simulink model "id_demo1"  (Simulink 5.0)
settings: Solver=ode45  SolverMode=SingleTasking  StartTime=0.0  StopTime=10  RelTol=1e-3  AbsTol=1e-3
libraries: simulink x1

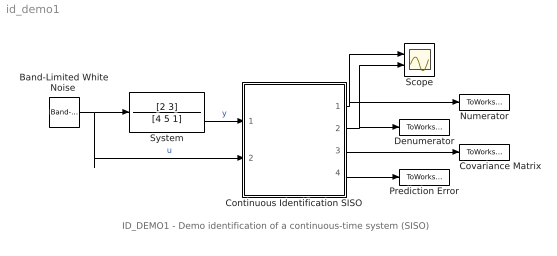
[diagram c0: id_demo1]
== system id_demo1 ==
  note: ID_DEMO1 - Demo identification of a continuous-time system (SISO)
  "Band-Limited White Noise " : simulink/Sources/Band-Limited White Noise  Cov=[0.1]  Ts=0.1  seed=[23341]
  Continuous Identification SISO : Subsystem  mask(Continuous Identification){par1=[1,2], tc=[0.5], par2=[0.985,0.01], poc=[0 0 0 0], kov=[10e6], ts=[1]}
      mask prompts: par1 "Degrees of numerator and denominator -  [dn, dd]:"; tc "Time constant of the filter - [Tc]:"; par2 "Exponential forgetting and Bittanti's correction - [L, d]:"; poc "Initial parameter estimates - [theta(1) ... theta(n)]:"; kov "Covariance matrix (see help, standard - [10e6]):"; ts "Sampling time - [ts]:"
      mask help: Continuous identification Authors: Lubos Cirka and Miroslav Fikar 1998 - 2006
      mask init:
      | % State-space realisation of continuous-time MIMO filters
      | %
      | % Input:
      | %    y1(t), ..., yn(t), u1(t), ..., um(t)
      | % Output:
      | %    y(t), y'(t), y''(t) ..., u(t), u'(t), ...
      | 
      | % Calculation of the denominator with multiple time constant tc
      | 
      | cit=par1(1);men=par1(2);L=par2(1);d=par2(2); n=cit+men+1;m=1;in=1;out=1;
      | den=1;
      | for i=1:men,
      |    den=conv([tc 1],den);
      | end;
      | a=fliplr(den(2:men+1)/den(1));
      | 
      | % State-space realisation of the output filter
      | 
      | A0=zeros(out*(men-1),out);
      | A1=eye(out*(men-1));
      | for i=1:men
      |    A2(1:out,out*(i-1)+1:i*out)=-a(i)*eye(out);
      | end
      | Ay=[A0 A1;A2];
      | B0=zeros(out*(men-1),out);
      | B1=eye(out,out);
      | By=[B0;B1];
      | 
      | C0=-eye(out*(men-1)+out);C0(1:out,1:out)=eye(out);
      | for i=1:men
      |    C1(1:out,out*(i-1)+1:i*out)=a(i)*eye(out);
      | end
      | Cy=[C0;C1]/den(1);
      | Dy=-[zeros(out,out);By]/den(1);
      | 
      | % State-space realisation of the input filter
      | 
      | a0=zeros(in*(men-1),in);
      | a1=eye(in*(men-1));
      | for i=1:men
      |    a2(1:in,in*(i-1)+1:i*in)=-a(i)*eye(in);
      | end
      | Au=[a0 a1;a2];
      | b0=zeros(in*(men-1),in);
      | b1=eye(in,in);
      | Bu=[b0;b1];
      | if cit==men
      |    c0=eye(in*(cit-1)+in);
      |    for i=1:cit
      |       c1(1:in,in*(i-1)+1:i*in)=-a(i)*eye(in);
      |    end
      |    Cu=[c0;c1]/den(1);
      |    Du=[zeros(in*(cit-1)+in,in);eye(in)]/den(1);
      | else
      |    c0=eye(in*(cit+1));
      |    c1=zeros(in*(cit+1),(men-cit-1)*in);
      |    Cu=[c0 c1]/den(1);
      |    Du=zeros(in*(cit+1),in);
      | end
  Covariance Matrix : ToWorkspace  VariableName=CovMatrix  SaveFormat=Array
  Denumerator : ToWorkspace  VariableName=A  SaveFormat=Array
  Numerator : ToWorkspace  VariableName=B  SaveFormat=Array
  Prediction Error : ToWorkspace  VariableName=PredError  SaveFormat=Array
  Scope : Scope  NumInputPorts=2
  System : TransferFcn  Numerator=[2 3]  Denominator=[4 5 1]
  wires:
  System/1 -> Continuous Identification SISO/1(y)  "y"
  "Band-Limited White Noise "/1 -> System/1, Continuous Identification SISO/2(u)  "u"
  Continuous Identification SISO/3("Covariance matrix ") -> Covariance Matrix/1
  Continuous Identification SISO/4(prediction error) -> Prediction Error/1
  Continuous Identification SISO/1(B) -> Numerator/1, Scope/1
  Continuous Identification SISO/2(A) -> Denumerator/1, Scope/2

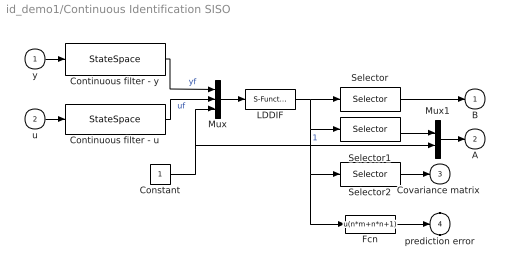
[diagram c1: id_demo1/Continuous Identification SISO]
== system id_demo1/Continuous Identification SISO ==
  y : Inport
  u : Inport  Port=2
  Constant : Constant
  Continuous filter - u : StateSpace  A=Au  B=Bu  C=Cu  D=Du
  Continuous filter - y : StateSpace  A=Ay  B=By  C=Cy  D=Dy
  Fcn : Fcn  Expr=u(n*m+n*n+1)
  LDDIF : S-Function  FunctionName=lddif_s  Parameters=m ,n+1 ,L ,d, [poc 0], kov, ts
  Mux : Mux  Inputs=3
  Mux1 : Mux  Inputs=2
  Selector : Selector  Elements=[men+cit+1:-1:men+1]  InputPortWidth=(n+1)*m+(n+1)*(n+1)+m
  Selector1 : Selector  Elements=[men:-1:1]  InputPortWidth=(n+1)*m+(n+1)*(n+1)+m
  Selector2 : Selector  Elements=[(n+1)*m+1:1:(n+1)*m+(n+1)*(n+1)]  InputPortWidth=(n+1)*m+(n+1)*(n+1)+m
  B : Outport  InitialOutput=0
  A : Outport  Port=2  InitialOutput=0
  "Covariance matrix " : Outport  Port=3  InitialOutput=0
  prediction error : Outport  Port=4  InitialOutput=0
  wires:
  LDDIF/1 -> Selector/1, Selector1/1, Selector2/1, Fcn/1
  Continuous filter - u/1 -> Mux/2  "uf"
  Continuous filter - y/1 -> Mux/1  "yf"
  u/1 -> Continuous filter - u/1
  y/1 -> Continuous filter - y/1
  Selector/1 -> B/1
  Mux/1 -> LDDIF/1
  Constant/1 -> Mux/3, Mux1/2  "1"
  Selector1/1 -> Mux1/1
  Mux1/1 -> A/1
  Selector2/1 -> "Covariance matrix "/1
  Fcn/1 -> prediction error/1
